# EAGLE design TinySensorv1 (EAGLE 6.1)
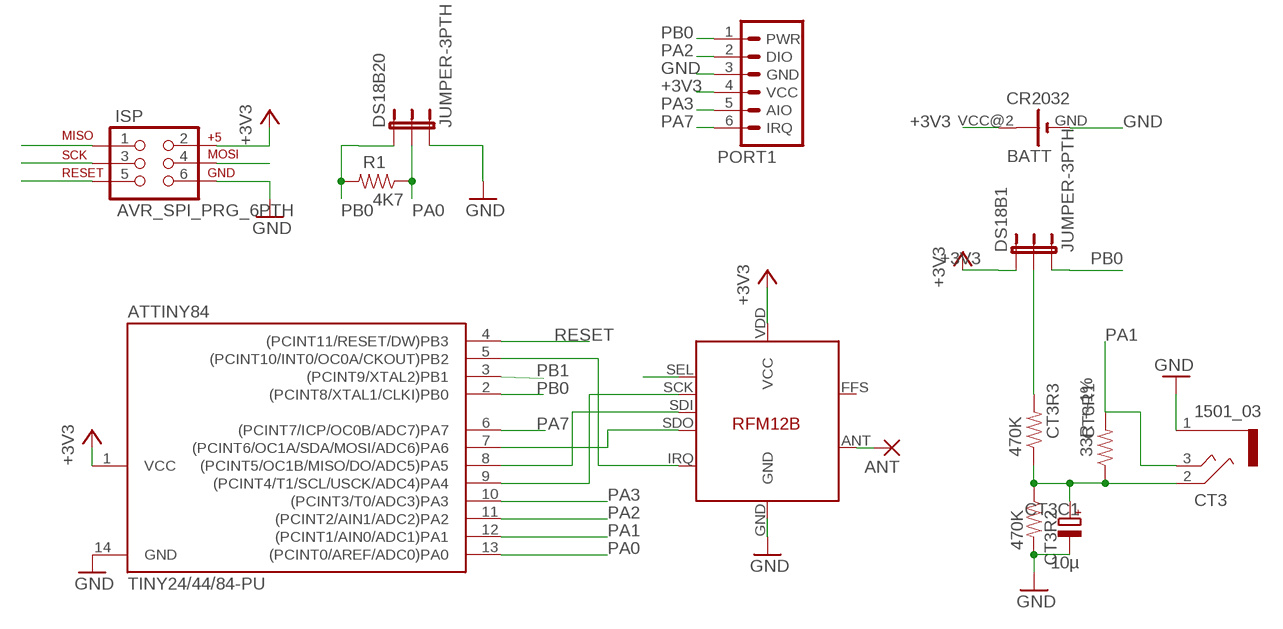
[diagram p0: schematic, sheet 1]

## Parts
ANT  1,6/0,8  [1,6/0,8]
ATTINY84  TINY24/44/84-PU  [DIL14]
BATT  CR2032  CR2032HCOMPACT  [BATT_CONN_CR2032]
CT3  1501_03  [1501_03]
CT3C1  10µ  CPOL-EUE1.8-4  [E1,8-4]
CT3R1  33R +-1%  RESISTORAXIAL-0.3  [AXIAL-0.3]
CT3R2  470K  RESISTORAXIAL-0.3  [AXIAL-0.3]
CT3R3  470K  RESISTORAXIAL-0.3  [AXIAL-0.3]
DS18B1  JUMPER-3PTH  [1X03]
DS18B20  JUMPER-3PTH  [1X03]
ISP  AVR_SPI_PRG_6PTH  [2X3]
PORT1  JEEPORT-FEMALE  [1X06_FEMALE_LOCK.010]
R1  4K7  RESISTORAXIAL-0.3  [AXIAL-0.3]
RFM12B  RFM12B  [RFM12B]

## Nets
+3V3 [power]: ATTINY84.1(VCC) BATT.VCC@2(+) DS18B1.1 ISP.2 PORT1.4(VCC) RFM12B.VDD(VCC)
GND [power]: ATTINY84.14(GND) BATT.GND(-) CT3.1 CT3C1.- CT3R2.P$2 DS18B20.3 ISP.6 PORT1.3(GND) RFM12B.GND
MISO: ATTINY84.8((PCINT5/OC1B/MISO/DO/ADC5)PA5) ISP.1 RFM12B.SDI
MOSI: ATTINY84.7((PCINT6/OC1A/SDA/MOSI/ADC6)PA6) ISP.4 RFM12B.SDO
N$1: CT3R3.P$2 DS18B1.2
N$6 [power]: ANT.1(P) RFM12B.ANT
N$10: CT3.2 CT3C1.+ CT3R1.P$1 CT3R2.P$1 CT3R3.P$1
PA0: ATTINY84.13((PCINT0/AREF/ADC0)PA0) DS18B20.2 R1.P$1
PA1: ATTINY84.12((PCINT1/AIN0/ADC1)PA1) CT3.3 CT3R1.P$2
PA2: ATTINY84.11((PCINT2/AIN1/ADC2)PA2) PORT1.2(DIO)
PA3: ATTINY84.10((PCINT3/T0/ADC3)PA3) PORT1.5(AIO)
PA7: ATTINY84.6((PCINT7/ICP/OC0B/ADC7)PA7) PORT1.6(IRQ)
PB0: ATTINY84.2((PCINT8/XTAL1/CLKI)PB0) DS18B1.3 DS18B20.1 PORT1.1(PWR) R1.P$2
PB1: ATTINY84.3((PCINT9/XTAL2)PB1) RFM12B.SEL
PB2: ATTINY84.5((PCINT10/INT0/OC0A/CKOUT)PB2) RFM12B.IRQ
RESET: ATTINY84.4((PCINT11/RESET/DW)PB3) ISP.5
SCK: ATTINY84.9((PCINT4/T1/SCL/USCK/ADC4)PA4) ISP.3 RFM12B.SCK
Unconnected: BATT.VCC@1(+) RFM12B.FFS

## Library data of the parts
ANT = JeeLabs:1,6/0,8: THROUGH-HOLE PAD
ATTINY84 = avr-7:TINY24/44/84
BATT = SnootLib:CR2032H: LI BATTERY CR2032
CT3 = con-lumberg:1501_03: Klinkensteckverbinder nach JISC 6560, 2,5 mm Jack connectors according to JISC 6560, 2.5 mm Source: http://www.lumberg.com/Produkte/PDFs/1501_03.pdf; OC_FARNELL: 1200127; OC_NEWARK: unknown
CT3C1 = resistor:CPOL-EU: POLARIZED CAPACITOR, European symbol
CT3R1-CT3R3 R1 = SparkFun:RESISTOR: Resistor
DS18B1 DS18B20 = SparkFun:JUMPER-3
ISP = SparkFun:AVR_SPI_PRG_6: AVR ISP 6 Pin This is the reduced ISP connector for AVR programming. Common on Arduino. This footprint will take up less PCB space and can be used with a 10-pin to 6-pin adapter such as SKU: BOB-08508
PORT1 = JeeParts:JEEPORT: PIN HEADER
RFM12B = JeeLabs:RFM12B

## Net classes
0 default: width 0.356 mm, drill 0.356 mm, clearance 0.356 mm
1 power: width 0.406 mm, drill 0.356 mm, clearance 0.406 mm

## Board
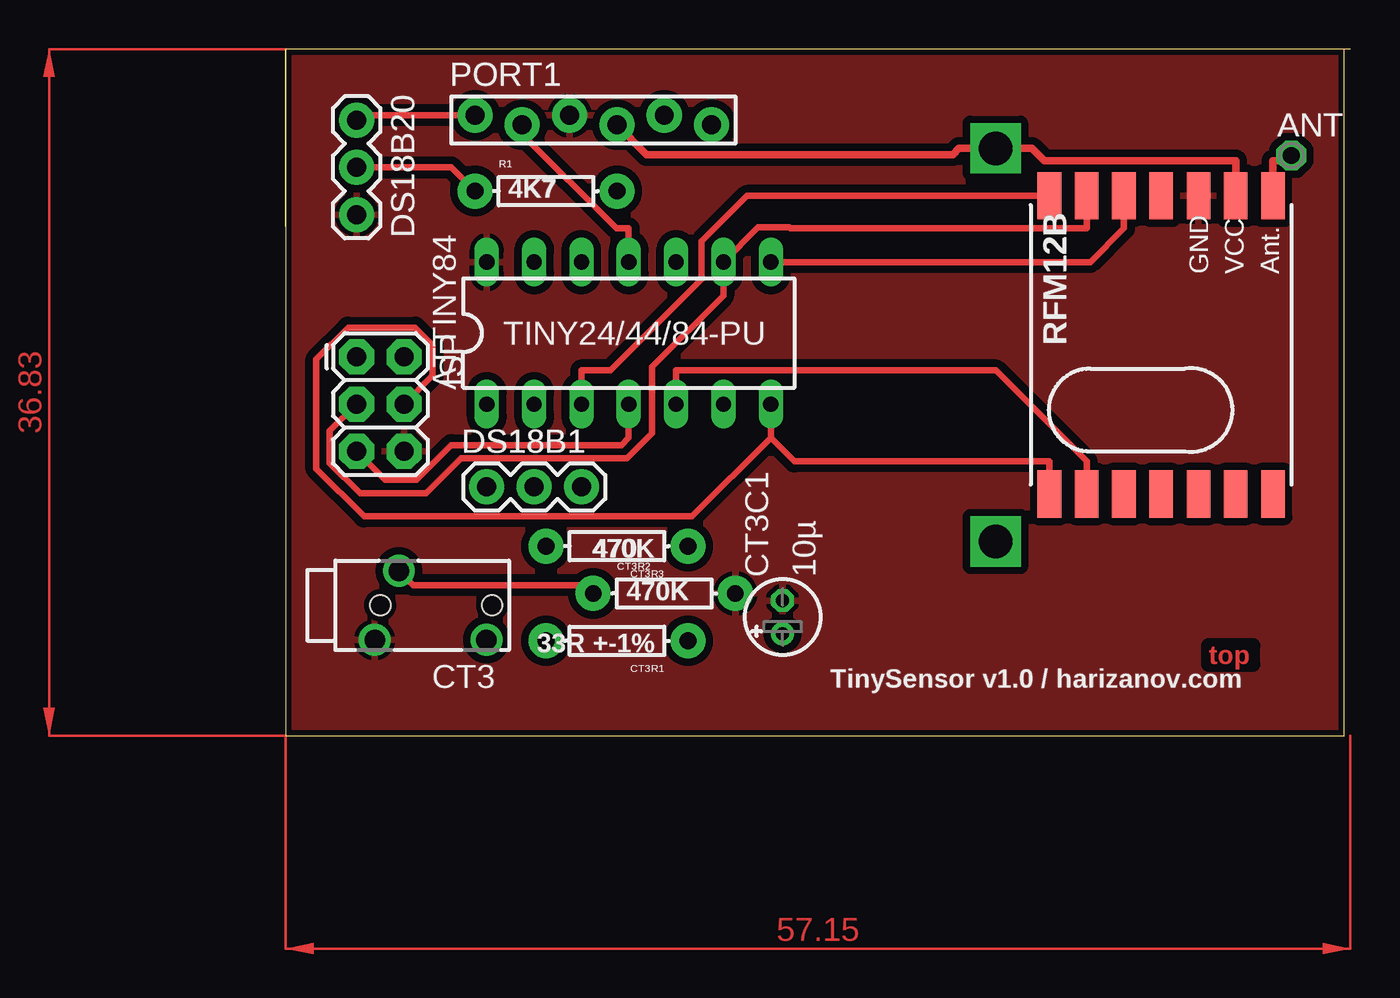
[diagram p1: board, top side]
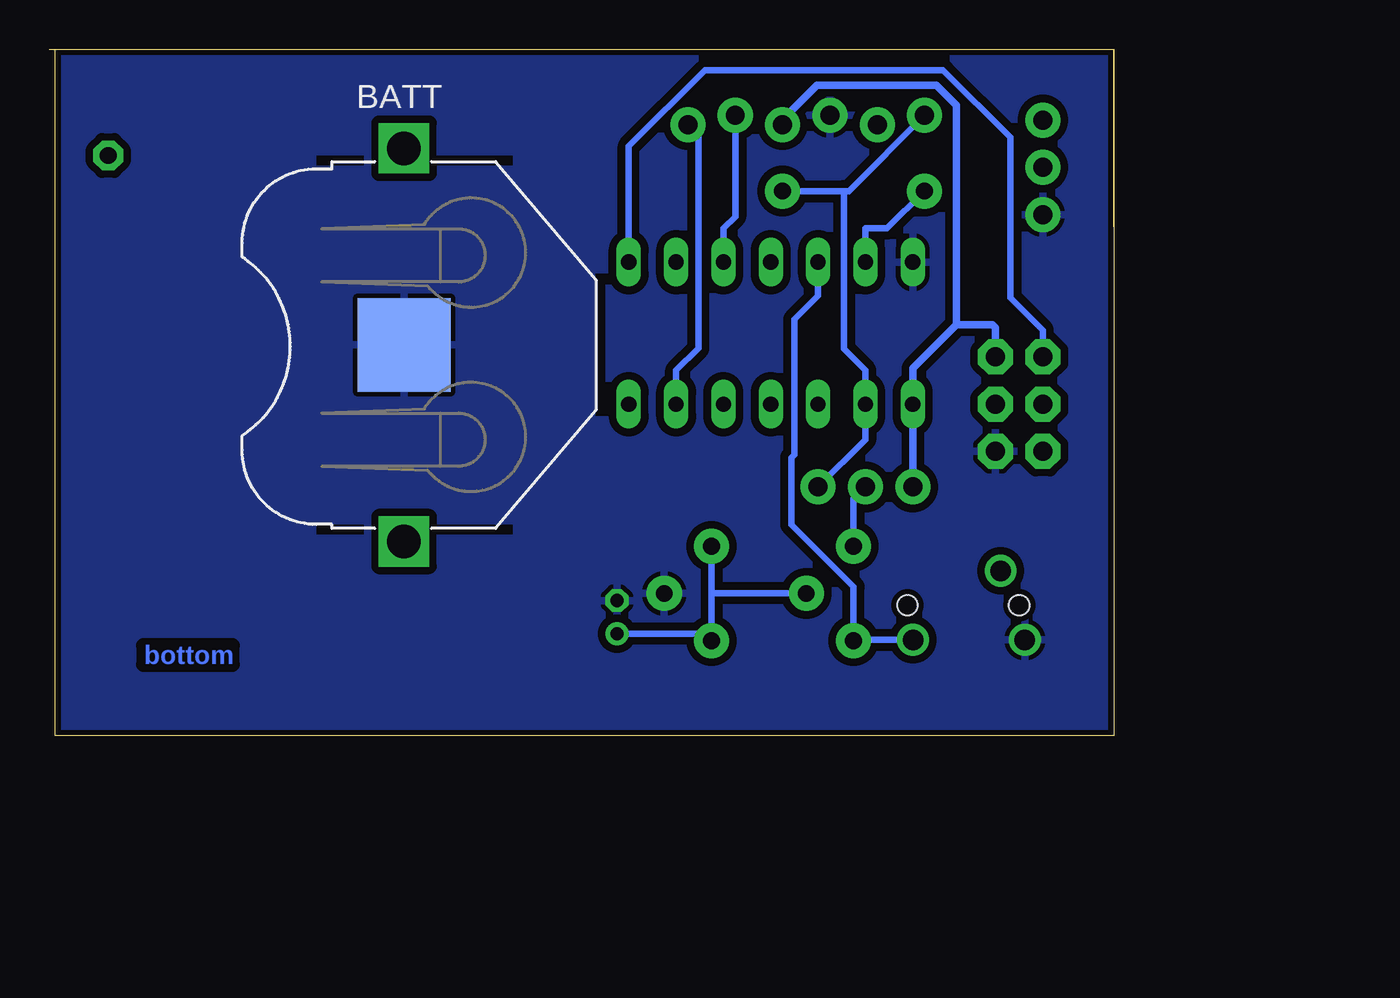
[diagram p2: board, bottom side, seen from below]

Size 57.15 x 36.83 mm. Coordinates in mm from the lower left corner, seen from the top.
Outline: 56.82,36.82 56.82,0 0,0 0,27.3
Outline: 0,27.3 0,36.83
Outline: 0,36.83 0,27.3
Outline: 57.15,36.83 0,36.83
Copper layers (1*16): Top 0.035mm / dielectric 1.5mm / Bottom 0.035mm
Design rules: minimum track width 12mil, minimum drill 24mil, track to track 10mil, track to pad 12mil, pad to pad 12mil, via to via 14mil, smd to smd 10mil, copper to edge 12mil, drill to drill 8mil, minimum pad ring 10mil, minimum via ring 8mil, stop-mask expansion 4mil, vias tented up to drill 0mil, thermal gap 10mil

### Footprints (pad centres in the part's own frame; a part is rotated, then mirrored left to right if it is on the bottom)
1,6/0,8 = drill 0.9 pad 1.6 octagon: 1 0,0
DIL14 = drill 0.813 long: 1 -7.62,-3.81; 2 -5.08,-3.81; 3 -2.54,-3.81; 4 0,-3.81; 5 2.54,-3.81; 6 5.08,-3.81; 7 7.62,-3.81; 8 7.62,3.81; 9 5.08,3.81; 10 2.54,3.81; 11 0,3.81; 12 -2.54,3.81; 13 -5.08,3.81; 14 -7.62,3.81
BATT_CONN_CR2032 = smd 5 x 5: GND 0,0 | drill 1.8 square: VCC@1 -10.55,0; VCC@2 10.55,0
1501_03 = drill 1.1 pad 1.7: 1 -1.85,0.3; 2 1.85,-1; 3 -1.85,-5.7 | hole 1.1: 0,0; 0,-6
E1,8-4 = drill 0.711 pad 1.168: + -0.889,0 | drill 0.711 pad 1.168 octagon: - 0.889,0
AXIAL-0.3 = drill 0.9 pad 1.88: P$1 -3.81,0; P$2 3.81,0
1X03 = drill 1.016 pad 1.88: 1 0,0; 2 2.54,0; 3 5.08,0
2X3 = drill 1.016 pad 1.88 octagon: 1 0,0; 2 0,2.54; 3 2.54,0; 4 2.54,2.54; 5 5.08,0; 6 5.08,2.54
1X06_FEMALE_LOCK.010 = drill 1.016 pad 1.88: 1 0,0.254; 2 2.54,-0.254; 3 5.08,0.254; 4 7.62,-0.254; 5 10.16,0.254; 6 12.7,-0.254
RFM12B = smd 2.54 x 1.27: ANT 8,-6; FFS -8,2; GND 8,-2; IRQ -8,4; P$8 -8,0; P$9 -8,-2; P$10 -8,-4; P$12 -8,-6; P$16 8,0; SCK 8,4; SDI 8,2; SDO -8,6; SEL 8,6; VDD 8,-4

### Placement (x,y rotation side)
ANT  53.98,31.11 0 top
ATTINY84  18.41,21.59 0 top
BATT  38.1,20.95 90 bottom
CT3  5.08,6.99 90 top
CT3C1  26.67,6.35 90 top
CT3R1  17.78,5.08 180 top
CT3R2  20.32,7.62 0 top
CT3R3  17.78,10.16 180 top
DS18B1  10.79,13.34 0 top
DS18B20  3.81,33.02 270 top
ISP  3.81,20.32 270 top
PORT1  10.16,33.02 0 top
R1  13.97,29.21 0 top
RFM12B  46.99,20.95 90 top

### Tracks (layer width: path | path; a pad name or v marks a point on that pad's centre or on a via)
+3V3
  Top 0.406: RFM12B.VDD 50.99,30.84 40.73,30.84 40.06,31.5 BATT.VCC@2 36.14,31.5 35.8,31.17 19.38,31.17 PORT1.4
  Bottom 0.406: 8.46,22.05 10.79,19.71 ATTINY84.1 DS18B1.1 | PORT1.4 17.78,33.02 15.92,34.88 9.52,34.88 8.46,33.82 8.46,22.05 | 8.46,22.05 6.53,22.05 6.35,21.87 ISP.2
GND
  pour Bottom: -1.27,38.1 58.42,38.1 58.42,-1.27 -1.27,-1.27
  pour Top: -2.54,39.37 60.96,39.37 60.96,-2.54 -2.54,-2.54
MISO
  Top 0.356: RFM12B.SDI 44.99,27.2 43.19,25.4 ATTINY84.8
  Bottom 0.356: ISP.1 3.81,21.74 5.56,23.5 5.56,32.1 9.16,35.7 21.94,35.7 26.04,31.61 ATTINY84.8
MOSI
  Top 0.356: 26.04,15.98 21.82,11.76 4.21,11.76 1.64,14.32 1.64,20.18 3.34,21.88 6.95,21.88 7.89,20.94 7.89,19.32 ISP.4 | 26.04,15.98 27.3,14.71 40.99,14.71 RFM12B.SDO | ATTINY84.7 26.04,15.98
N$1
  Bottom 0.356: DS18B1.2 13.97,12.7 CT3R3.P$2
N$6
  Top 0.406: RFM12B.ANT 52.99,30.84 53.7,30.84 ANT.1
N$10
  Top 0.356: CT3R2.P$1 16.06,8.07 6.85,8.07 CT3.2
  Bottom 0.356: 21.59,5.46 CT3R1.P$1 | 21.59,7.62 21.59,5.46 | 21.59,5.46 CT3C1.+ | CT3R3.P$1 21.59,7.62 | CT3R2.P$1 21.59,7.62
PA0
  Top 0.356: DS18B20.2 8.89,30.48 R1.P$1
  Bottom 0.356: ATTINY84.13 13.34,27.2 12.17,27.2 R1.P$1
PA1
  Bottom 0.356: 13.97,5.13 13.97,7.98 17.31,11.32 17.31,14.9 17.14,15.07 17.14,22.33 15.88,23.6 ATTINY84.12 | CT3R1.P$2 13.97,5.13 | 13.97,5.13 CT3.3
PA2
  Top 0.356: ATTINY84.11 18.41,27.2 17.76,27.2 12.7,32.27 PORT1.2
PA3
  Bottom 0.356: ATTINY84.10 20.95,27.2 20.32,27.84 PORT1.5
PA7
  Bottom 0.356: ATTINY84.6 23.5,19.58 22.3,20.77 22.3,32.21 PORT1.6
PB0
  Top 0.356: PORT1.1 4.06,33.27 DS18B20.1
  Bottom 0.356: 14.49,29.21 14.22,29.21 PORT1.1 | R1.P$2 14.49,29.21 | 14.49,29.21 14.49,20.74 13.34,19.58 ATTINY84.2 13.34,15.88 DS18B1.3
PB1
  Top 0.356: ATTINY84.3 15.88,19.58 17.43,19.58 22.32,24.48 22.32,26.51 24.77,28.95 RFM12B.SEL
PB2
  Top 0.356: ATTINY84.5 20.95,19.58 38.11,19.58 42.99,14.71 RFM12B.IRQ
RESET
  Top 0.356: ATTINY84.4 18.41,15.98 18.02,15.58 8.89,15.58 7.02,13.71 5.34,13.71 ISP.5
SCK
  Top 0.356: RFM12B.SCK 42.99,27.2 27.11,27.2 27.05,27.26 25.35,27.26 ATTINY84.9 23.5,23.6 19.67,19.77 19.67,16.21 18.33,14.87 9.4,14.87 7.53,12.99 3.99,12.99 2.37,14.61 2.37,16.34 ISP.3
(copper drawn outside any net)
  shapes: Top area x2

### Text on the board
Top: top
Bottom: bottom
_tsilk: PORT1 | DS18B20 | ANT | R1 | 4K7 | GND | VCC | Ant. | ISP | TINY24/44/84-PU | RFM12B | DS18B1 | 470K | CT3R2 | CT3R3 | 10µ | 470K | 33R +-1% | CT3R1 | TinySensor v1.0 / harizanov.com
